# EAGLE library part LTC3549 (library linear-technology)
250mA Low VIN Buck Source: http://www.linear.com/pc/downloadDocument.do?navId=H0,C1,C1003,C1042,C1032,C1063,P26952,D16357
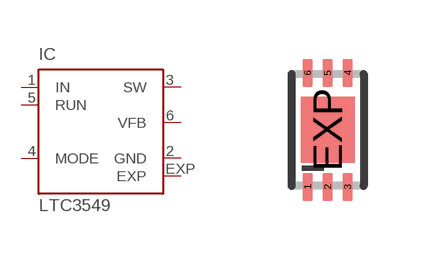
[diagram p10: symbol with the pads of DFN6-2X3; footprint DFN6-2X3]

Designator prefix IC

## LTC3549 (MPN: LTC3549EDCB#TRMPBF; OC_FARNELL: 1715241; OC_NEWARK: 56M8010)  [DFN6-2X3]
1  IN  in
2  GND  pwr
3  SW  out
4  MODE  in
5  RUN  in
6  VFB  in
EXP  EXP  pas

## Footprint DFN6-2X3 (pad centres in mm)
DCB Package 6-Lead Plastic DFN (2mm × 3mm) Source: http://www.linear.com/pc/downloadDocument.do?navId=H0,C1,C1003,C1042,C1032,C1063,P26952,D16357
smd 0.25 x 0.7: 1 -0.5,-1.425; 2 0,-1.425; 3 0.5,-1.425; 4 0.5,1.425; 5 0,1.425; 6 -0.5,1.425
smd 1.35 x 1.65: EXP 0,0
